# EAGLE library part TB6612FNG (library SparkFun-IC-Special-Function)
Toshiba 1A dual motor driver IC-09363
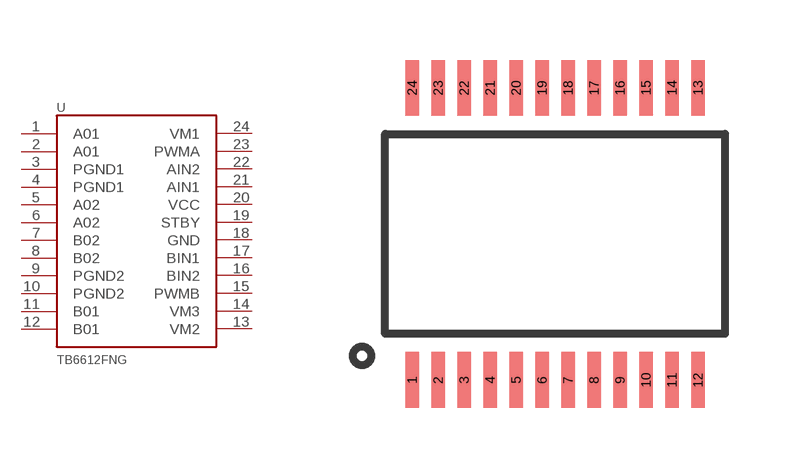
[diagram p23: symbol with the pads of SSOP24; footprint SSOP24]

Designator prefix -

## TB6612FNG (PROD_ID: IC-09363; VALUE: TB6612FNG)  [SSOP24]
1  A01
2  A01
3  PGND1
4  PGND1
5  A02
6  A02
7  B02
8  B02
9  PGND2
10  PGND2
11  B01
12  B01
13  VM2
14  VM3
15  PWMB
16  BIN2
17  BIN1
18  GND
19  STBY
20  VCC
21  AIN1
22  AIN2
23  PWMA
24  VM1

## Footprint SSOP24 (pad centres in mm)
smd 0.348 x 1.397: 1 -3.575,-3.656; 2 -2.925,-3.656; 3 -2.275,-3.656; 4 -1.625,-3.656; 5 -0.975,-3.656; 6 -0.325,-3.656; 7 0.325,-3.656; 8 0.975,-3.656; 9 1.625,-3.656; 10 2.275,-3.656; 11 2.925,-3.656; 12 3.575,-3.656; 13 3.575,3.656; 14 2.925,3.656; 15 2.275,3.656; 16 1.625,3.656; 17 0.975,3.656; 18 0.325,3.656; 19 -0.325,3.656; 20 -0.975,3.656; 21 -1.625,3.656; 22 -2.275,3.656; 23 -2.925,3.656; 24 -3.575,3.656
